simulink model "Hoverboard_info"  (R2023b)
settings: Solver=VariableStepAuto  StartTime=0.0  StopTime=10  RelTol=1e-3
libraries: simulink_extras x1

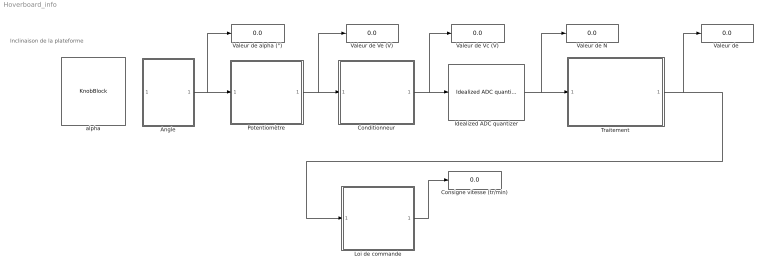
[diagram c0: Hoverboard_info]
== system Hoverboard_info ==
  note: Inclinaison de la plateforme
  Angle : Subsystem
  Conditionneur : Subsystem  mask{K=27/4, Vo=115/54}
      mask prompts: K "Gain (pente) K :"; Vo "Ordonnée à l'origine (V) Vo :"
  Consigne vitesse (tr/min) : Display
  Idealized ADC quantizer : simulink_extras/Additional Discrete/Idealized ADC quantizer  NumberOfConverterBits=1  Vmin=1  Vmax=3  OutputDataType=int16  OutputNegativeValues=off
  Loi de commande : Subsystem
  Potentiomètre : Subsystem
  Traitement : Subsystem  mask{q=1, No=0}
      mask prompts: q "Facteur d'échelle q :"; No "Décalage No :"
  "Valeur de " : Display
  Valeur de N : Display
  Valeur de Vc (V) : Display
  Valeur de Ve (V) : Display
  Valeur de alpha (°) : Display
  alpha : KnobBlock  LabelPosition=Hide  ScaleMin=-20  ScaleMax=20
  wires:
  Angle/1(Out1) -> Valeur de alpha (°)/1, Potentiomètre/1(In1)
  Conditionneur/1(Out1) -> Idealized ADC quantizer/1, Valeur de Vc (V)/1
  Potentiomètre/1(Out1) -> Conditionneur/1(In1), Valeur de Ve (V)/1
  Idealized ADC quantizer/1 -> Valeur de N/1, Traitement/1(In1)
  Traitement/1(Out1) -> "Valeur de "/1, Loi de commande/1(In1)
  Loi de commande/1(Out1) -> Consigne vitesse (tr/min)/1

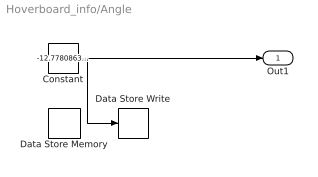
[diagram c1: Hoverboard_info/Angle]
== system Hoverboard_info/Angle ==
  Constant : Constant  Value=-12.77808634440104
  Data Store Memory : DataStoreMemory  DataStoreName=alpha  WriteAfterWriteMsg=warning  ShowAdditionalParam=off
  Data Store Write : DataStoreWrite  DataStoreName=alpha  IndexOptions=Index vector (dialog)  Indices=1  OutputSizes=1
  Out1 : Outport
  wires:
  Constant/1 -> Out1/1, Data Store Write/1

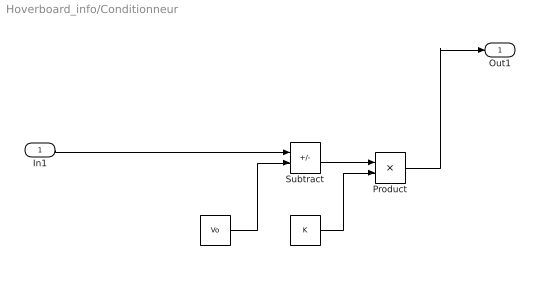
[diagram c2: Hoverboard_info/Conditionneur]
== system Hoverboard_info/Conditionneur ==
  In1 : Inport
  " " : Constant  Value=K
  "  " : Constant  Value=Vo
  Product : Product
  Subtract : Sum  Inputs=+-
  Out1 : Outport
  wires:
  Subtract/1 -> Product/1
  " "/1 -> Product/2
  "  "/1 -> Subtract/2
  Product/1 -> Out1/1
  In1/1 -> Subtract/1

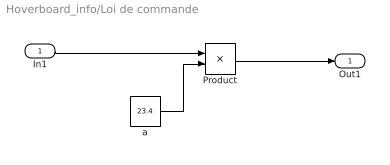
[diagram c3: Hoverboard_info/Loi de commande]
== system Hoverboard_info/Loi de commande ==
  In1 : Inport
  Product : Product
  a : Constant  Value=23.4
  Out1 : Outport
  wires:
  a/1 -> Product/2
  In1/1 -> Product/1
  Product/1 -> Out1/1

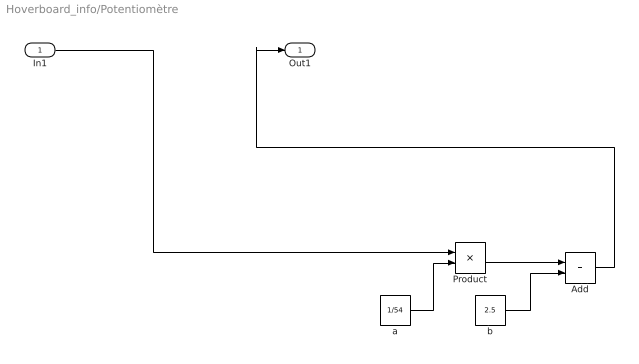
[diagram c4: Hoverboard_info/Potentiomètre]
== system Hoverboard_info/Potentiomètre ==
  In1 : Inport
  Add : Sum
  Product : Product
  a : Constant  Value=1/54
  b : Constant  Value=2.5
  Out1 : Outport
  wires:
  a/1 -> Product/2
  Product/1 -> Add/1
  In1/1 -> Product/1
  Add/1 -> Out1/1
  b/1 -> Add/2

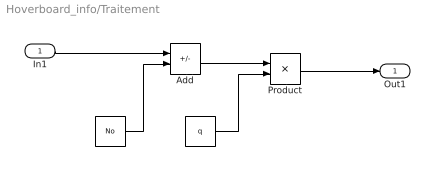
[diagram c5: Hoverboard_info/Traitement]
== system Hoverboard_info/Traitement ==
  In1 : Inport
  " " : Constant  Value=No
  "   " : Constant  Value=q
  Add : Sum  Inputs=+-
  Product : Product
  Out1 : Outport
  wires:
  Product/1 -> Out1/1
  "   "/1 -> Product/2
  Add/1 -> Product/1
  " "/1 -> Add/2
  In1/1 -> Add/1
